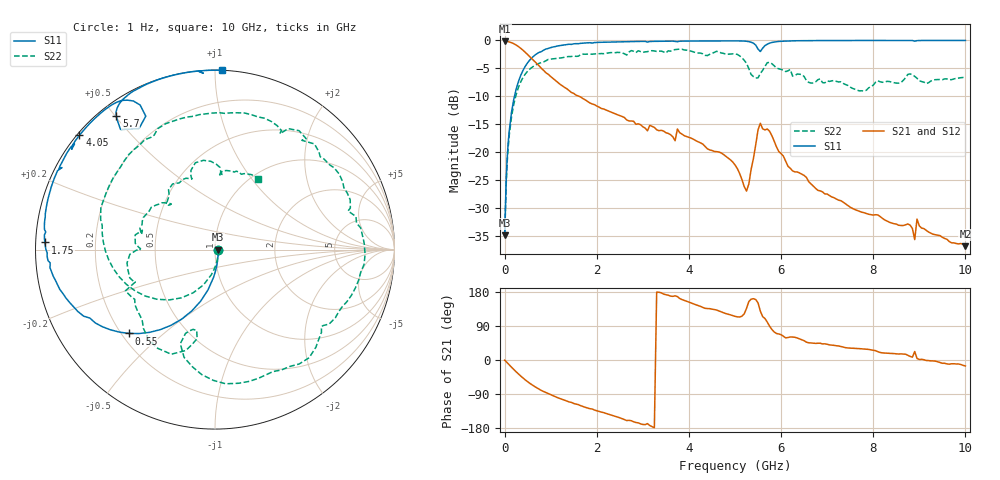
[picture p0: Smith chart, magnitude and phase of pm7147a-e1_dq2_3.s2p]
# GHz S DB R 50
! S-Parameters data
! Freq  dbS11  angS11  dbS21  angS21  dbS12  angS12  dbS22  angS22
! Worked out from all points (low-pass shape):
!   279 points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, 1 Hz to 10 GHz, reference 50 ohm
!   highest |S21| = -0.16 dB at 25.12 kHz (marker M1); lowest = -36.9 dB at 10 GHz (marker M2)
!   |S21| within 3 dB of the highest: start of sweep to 577.2 MHz
!   lowest |S11| = -34.9 dB at 25.12 kHz (marker M3), VSWR 1.04, Z = 51.8 - j0.00365 ohm
!   |S11| at or under -10 dB: start of sweep to 214.3 MHz
!   |S22| runs from -34.9 to -1.5 dB; largest |S21 - S12| = 0
!   S11 on the Smith chart (normalised r, x): 1 Hz: 1.04, -0.00; 550 MHz: 0.23, -0.39; 1.75 GHz: 0.03, +0.02; 4.05 GHz: 0.01, +0.37; 5.7 GHz: 0.05, +0.50; 10 GHz: 0.00, +1.04
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1e-09  -34.88 -0.0  -0.16 0.0  -0.16 0.0  -34.88 -0.0
2.51189e-05  -34.89 -0.1  -0.16 -0.0  -0.16 -0.0  -34.89 -0.1
0.05011872  -22.01 -81.5  -0.19 -6.4  -0.19 -6.4  -22.73 -83.3
0.15  -12.85 -99.8  -0.40 -19.0  -0.40 -19.0  -13.67 -108.2
0.55  -3.47 -135.9  -2.93 -61.8  -2.93 -61.8  -5.11 -164.3
0.95  -1.42 -157.8  -6.08 -88.7  -6.08 -88.7  -3.38 159.9
1.7  -0.48 178.7  -10.41 -122.8  -10.41 -122.8  -2.46 111.3
1.75  -0.46 177.6  -10.64 -124.8  -10.64 -124.8  -2.47 108.1
2.75  -0.20 158.4  -14.43 -160.3  -14.43 -160.3  -1.82 54.7
3.35  -0.15 149.3  -16.16 178.8  -16.16 178.8  -1.92 23.1
4.05  -0.11 139.8  -17.51 150.5  -17.51 150.5  -1.92 -18.5
4.55  -0.08 133.3  -19.88 133.1  -19.88 133.1  -2.13 -44.1
5.05  -0.08 126.4  -22.93 113.8  -22.93 113.8  -2.50 -85.5
5.25  -0.15 122.7  -26.98 136.3  -26.98 136.3  -4.10 -106.0
5.5  -1.54 117.4  -16.01 150.7  -16.01 150.7  -6.70 -102.7
5.7  -0.68 126.5  -15.86 100.0  -15.86 100.0  -3.99 -112.7
6.2  -0.08 118.7  -22.90 60.7  -22.90 60.7  -5.20 -155.3
6.7  -0.03 113.2  -26.10 44.3  -26.10 44.3  -7.64 179.3
8.35  -0.01 98.9  -32.57 17.6  -32.57 17.6  -7.35 112.2
8.9  -0.13 93.8  -35.67 22.4  -35.67 22.4  -6.44 89.2
8.95  -0.03 95.2  -32.01 4.1  -32.01 4.1  -6.77 86.5
10  -0.00 87.8  -36.85 -15.7  -36.85 -15.7  -6.75 58.8
